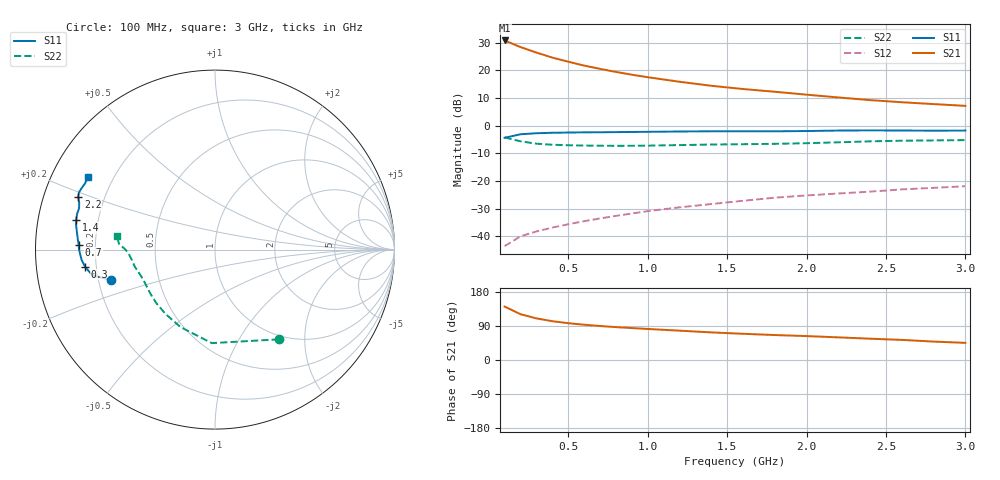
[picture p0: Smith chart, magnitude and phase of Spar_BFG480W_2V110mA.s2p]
! Filename: 2110BFG480.001
! Title: BFG480W
! Bias: Vce=2V; Ic=110mA
! Company: NXP Semiconductors NL
! User: Quality&Reliability T&D
! Measure time: 10 Nov 1999 / 11:55:13
#  MHz  S  MA  R 50
! Freq  S11  S21  S12  S22  :
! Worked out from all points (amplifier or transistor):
!   20 points, 100 MHz to 3 GHz, reference 50 ohm
!   highest |S21| = 30.9 dB at 100 MHz (marker M1)
!   |S21| within 3 dB of that: start of sweep to 230.2 MHz
!   unconditionally stable (mu >= 1): 497.9 MHz to end of sweep
!   at 400 MHz: K = 0.94, MSG = 30.8 dB, |S12| = -36.9 dB
!   at 1.2 GHz: K = 1.13, MAG = 20.6 dB, |S12| = -29.6 dB
!   at 3 GHz: K = 1.13, MAG = 12.4 dB, |S12| = -21.9 dB
!   S11 on the Smith chart (normalised r, x): 100 MHz: 0.25, -0.14; 300 MHz: 0.16, -0.06; 700 MHz: 0.14, +0.02; 1.4 GHz: 0.12, +0.10; 2.2 GHz: 0.10, +0.18; 3 GHz: 0.11, +0.26
100  0.6035 -163.6  34.9 141.0  0.006595 65.5  0.6133 -54.6
200  0.6998 -168.3  26.47 120.8  0.009946 58.6  0.5214 -91.9
300  0.7301 -172.5  21.08 109.8  0.01218 58.9  0.4726 -113.9
400  0.745 -175.5  17.11 102.4  0.0143 61.2  0.452 -127.6
500  0.7519 -178.0  14.4 97.2  0.01645 63.6  0.4428 -137.0
600  0.7574 179.8  12.27 93.1  0.01867 65.5  0.4372 -143.5
700  0.7602 178.0  10.69 89.7  0.02095 67.6  0.4339 -148.5
800  0.7649 176.2  9.408 86.8  0.0233 69.0  0.4323 -152.7
900  0.77 174.5  8.375 84.3  0.02568 70.6  0.4329 -156.1
1000  0.775 172.9  7.553 81.9  0.02835 71.4  0.4356 -159.2
1200  0.7853 170.2  6.244 77.4  0.03327 72.7  0.4455 -164.0
1400  0.791 167.9  5.281 72.9  0.03813 73.3  0.456 -167.6
1600  0.7936 165.6  4.613 69.2  0.04371 73.8  0.4621 -170.6
1800  0.7917 163.0  4.116 65.8  0.04971 74.0  0.4698 -173.8
2000  0.8005 160.9  3.643 63.1  0.05465 74.6  0.4818 -177.3
2200  0.8167 158.9  3.245 59.7  0.05922 74.2  0.5003 179.8
2400  0.8222 157.1  2.906 56.2  0.06404 73.6  0.5207 177.9
2600  0.8183 155.3  2.658 53.0  0.07031 72.7  0.535 176.7
2800  0.8126 152.9  2.461 48.6  0.07493 71.2  0.5414 174.9
3000  0.8166 150.3  2.285 45.2  0.08025 70.3  0.5484 172.2
